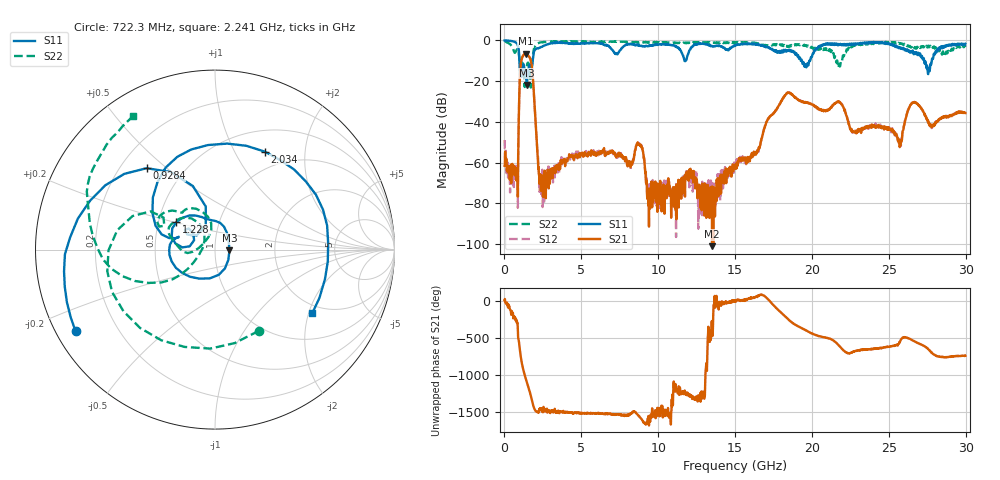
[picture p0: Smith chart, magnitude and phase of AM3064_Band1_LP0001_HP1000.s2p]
# Hz S DB R 50.0
!freq dBS11 angS11 dBS21 angS21 dBS12 angS12 dBS22 angS22
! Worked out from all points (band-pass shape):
!   1600 points, 10 MHz to 29.98 GHz, reference 50 ohm
!   highest |S21| = -6.48 dB at 1.397 GHz (marker M1); lowest = -101.0 dB at 13.51 GHz (marker M2)
!   |S21| within 3 dB of the highest: 1.112 GHz to 1.699 GHz (587 MHz wide, 41.8 % of centre)
!   lowest |S11| = -21.9 dB at 1.453 GHz (marker M3), VSWR 1.18, Z = 58.8 - j0.511 ohm
!   |S11| at or under -10 dB: 973.5 MHz to 1.831 GHz (857.7 MHz wide, 61.2 % of centre); 19.35 GHz to 19.82 GHz (469.8 MHz wide, 2.4 % of centre); 27.3 GHz to 27.79 GHz (496.4 MHz wide, 1.8 % of centre)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
!   |S22| runs from -23.1 to -0.2 dB; largest |S21 - S12| = 0.0059
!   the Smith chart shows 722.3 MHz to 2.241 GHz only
!   S11 on the Smith chart (normalised r, x): 722.3 MHz: 0.06, -0.27; 928.4 MHz: 0.31, +0.43; 1.228 GHz: 0.62, +0.21; 2.034 GHz: 0.76, +1.33; 2.241 GHz: 1.74, -2.12
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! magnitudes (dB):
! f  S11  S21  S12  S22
! 10 MHz  0.0  -61.6  -48.9  -0.2
! 722.3 MHz  -0.9  -66.6  -63.7  -5.8
! 928.4 MHz  -4.5  -39.7  -39.7  -6.1
! 1.228 GHz  -11.5  -7.4  -7.3  -13.1
! 1.397 GHz  -17.2  -6.5  -6.5  -15.1
! 1.453 GHz  -21.9  -6.6  -6.6  -12.7
! 1.753 GHz  -13.4  -11.3  -11.2  -17.2
! 2.034 GHz  -4.3  -41.1  -41.1  -2.1
! 2.241 GHz  -3.8  -65.9  -65.3  -1.2
! 5.015 GHz  -1.4  -55.7  -55.3  -0.8
! 8.763 GHz  -2.6  -50.9  -51.1  -1.1
! 9.344 GHz  -2.7  -72.9  -69.5  -0.9
! 10 GHz  -2.0  -71.7  -74.7  -0.9
! 13.51 GHz  -2.8  -101.0  -75.9  -1.1
! 15 GHz  -2.6  -62.9  -61.2  -1.3
! 18.34 GHz  -5.5  -26.1  -26.1  -2.7
! 19.99 GHz  -8.1  -31.4  -31.5  -3.4
! 25 GHz  -1.4  -42.6  -43.1  -1.1
! 25.73 GHz  -3.4  -51.8  -52.3  -1.7
! 26.63 GHz  -6.8  -30.6  -30.4  -3.1
! 27.56 GHz  -16.6  -39.8  -39.6  -2.8
! 29.98 GHz  -1.7  -35.7  -35.1  -3.2
